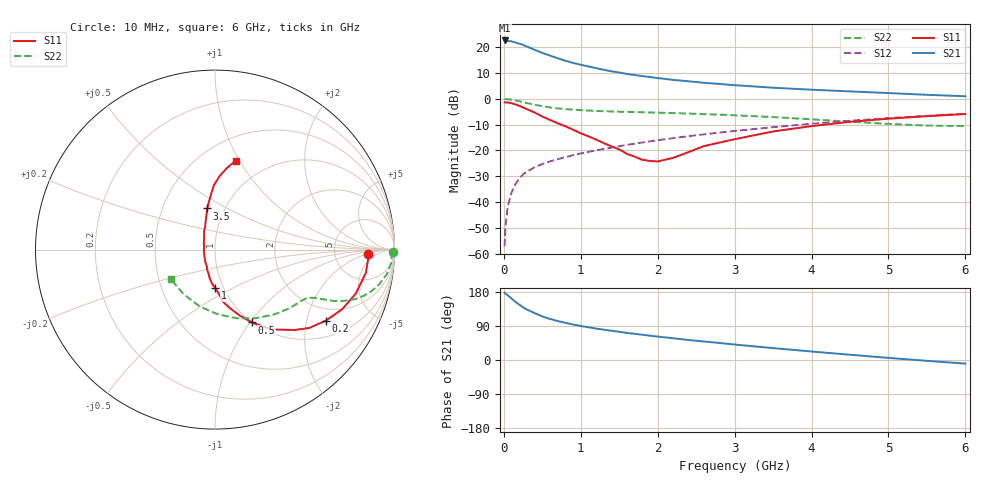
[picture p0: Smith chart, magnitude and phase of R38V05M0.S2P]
! SIEMENS Small Signal Semiconductors
! BFR181
! Si NPN RF Bipolar Junction Transistor in SOT23
! VCE = 8 V  IC = 5 mA
! Common Emitter S-Parameters:  May  1996
# GHz  S  MA  R  50
!  f  S11  S21  S12  S22
! GHz  MAG  ANG  MAG  ANG  MAG  ANG  MAG  ANG
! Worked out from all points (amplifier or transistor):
!   36 points, 10 MHz to 6 GHz, reference 50 ohm
!   highest |S21| = 22.6 dB at 10 MHz (marker M1)
!   |S21| within 3 dB of that: start of sweep to 351.2 MHz
!   unconditionally stable (mu >= 1): 1.209 GHz to 3.113 GHz
!   at 250 MHz: K = 0.40, MSG = 25.1 dB, |S12| = -29.3 dB
!   at 1.4 GHz: K = 1.04, MAG = 13.6 dB, |S12| = -18.9 dB
!   at 6 GHz: K = 0.86, MSG = 3.4 dB, |S12| = -5.8 dB
!   lowest NFmin = 1.55 dB at 450 MHz
!   S11 on the Smith chart (normalised r, x): 10 MHz: 12, -2; 200 MHz: 1.53, -2.62; 500 MHz: 1.00, -1.02; 1 GHz: 0.92, -0.41; 3.5 GHz: 0.83, +0.40; 6 GHz: 0.72, +0.96
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0.01  0.8526 -1.7  13.54 177.5  0.0014 91.7  0.9909 -0.8
0.02  0.8549 -3.5  13.34 175.7  0.0033 86.4  0.9854 -1.7
0.05  0.8507 -8.7  13.21 170.8  0.0081 83.8  0.9847 -4.3
0.1  0.8221 -17.3  13.02 162.4  0.0153 80.6  0.9666 -8.2
0.15  0.7827 -25.1  12.33 153.4  0.0222 76.1  0.9347 -12.0
0.2  0.7339 -32.6  11.74 146.2  0.0285 73.2  0.9018 -14.9
0.25  0.6832 -39.7  11.11 139.0  0.0344 70.3  0.8653 -17.4
0.3  0.6302 -45.3  10.32 133.1  0.0389 68.4  0.8298 -19.4
0.4  0.5442 -54.8  8.936 123.8  0.0473 65.5  0.7701 -21.8
0.5  0.455 -63.1  7.776 114.9  0.0547 64.4  0.722 -23.4
0.6  0.3907 -69.6  6.898 108.4  0.0615 64.1  0.6825 -24.2
0.7  0.3373 -75.6  6.136 102.9  0.0677 63.5  0.6541 -24.9
0.8  0.2947 -81.2  5.49 98.0  0.0742 63.3  0.6337 -25.3
1  0.2155 -89.4  4.579 89.8  0.0875 63.8  0.6053 -26.3
1.1  0.1881 -95.4  4.245 86.4  0.0939 63.8  0.5938 -26.9
1.6  0.0862 -129.4  3.045 71.5  0.1285 63.8  0.5596 -30.6
1.9  0.0627 -172.7  2.651 64.1  0.1501 63.2  0.5444 -33.9
2.2  0.0718 150.1  2.331 57.4  0.1732 62.1  0.5308 -37.5
3.5  0.2335 100.6  1.643 31.4  0.2829 53.3  0.4435 -59.6
4.5  0.3596 90.9  1.395 13.9  0.3773 43.4  0.3605 -87.6
5.5  0.4628 81.4  1.198 -2.2  0.4702 31.3  0.3038 -125.2
6  0.5086 76.8  1.124 -9.5  0.5142 24.5  0.2964 -146.4
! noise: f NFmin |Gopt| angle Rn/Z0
0.45  1.55  0.48  17  0.36
0.9  1.65  0.4  35  0.34
1.8  2  0.18  88  0.34
